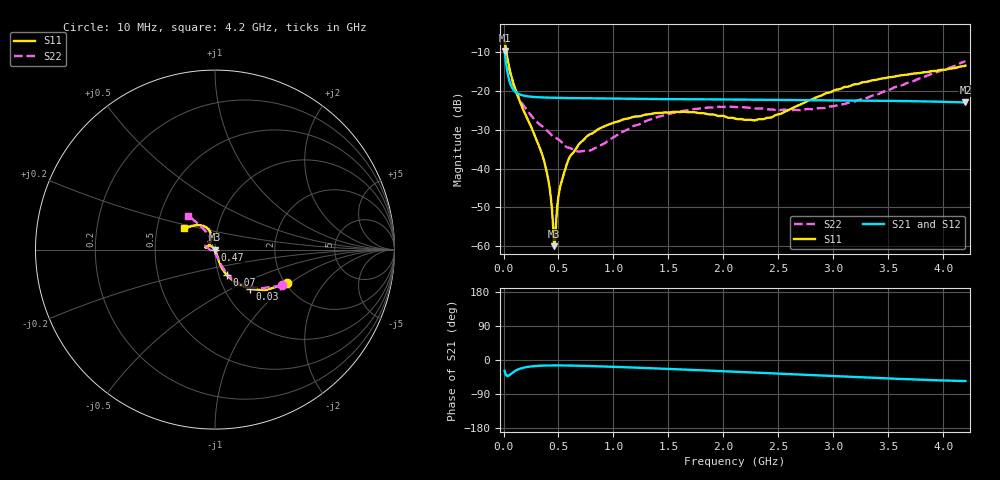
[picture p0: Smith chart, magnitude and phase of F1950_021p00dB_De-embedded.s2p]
! Integrated Device Technology
! Corporate Headquarters
! 6024 Silver Creek Valley Road
! San Jose, CA 95138  USA
! Phone:  1-408-284-8200
! Toll Free:  1-800-223-1366
! Webpage:  http://www.idt.com/
! Timing and RF Division
! 515 Groton Road, Suite 102
! Westford, MA 01886-6024
! Device:  F1950
! Description: 7-bit 0.25 dB Digital Step Attenuator
! Frequency:  150.0 -  4000.00 MHz
! Package:  4x4 mm Thin QFN Plastic Package: 24 pin
! Ports:  2 RF, 12 DC
!  Pin  1  = D0
!  Pin  2  = VDD
!  Pin  3  = Vmode
!  Pin  4  = GND
!  Pin  5  = RF1  =  Port 1
!  Pin  6  = GND
!  Pin  7  = GND
!  Pin  8  = GND
!  Pin  9  = GND
!  Pin 10  = GND
!  Pin 11  = GND
!  Pin 12  = GND
!  Pin 13  = GND
!  Pin 14  = RF2  =  Port 2
!  Pin 15  = GND
!  Pin 16  = LE
!  Pin 17  = CLK
!  Pin 18  = DATE
!  Pin 19  = D6
!  Pin 20  = D5
!  Pin 21  = D4
!  Pin 22  = D3
!  Pin 23  = D2
!  Pin 24  = D1
! State:  84
! Atten State:  21.00 dB
! Voltage:  +5.00 Volts
! Current:  Not Measured mA
! Data:  The device was measured on a the F195X evaluation board which has
!  individual transmission lines to the RF pins.  Data was collected
!  using a calibrated network analyzer.  The evaluation board was
!  de-embedded using a TRL calibration technique.
!  The reference plane is the edge of the package pin.
! Misc:  Board 2019
!  Action Tracker AT0250
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# GHz S dB R 50
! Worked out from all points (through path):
!   420 points, 10 MHz to 4.2 GHz, reference 50 ohm
!   highest |S21| = -9.63 dB at 10 MHz (marker M1); lowest = -23.0 dB at 4.2 GHz (marker M2)
!   group delay of S21, straight-line fit = 28.2 ps
!   lowest |S11| = -60.0 dB at 460 MHz (marker M3), VSWR 1.00, Z = 49.9 - j0.0787 ohm
!   |S11| at or under -10 dB: 26.17 MHz to end of sweep
!   |S22| runs from -35.6 to -7.5 dB; largest |S21 - S12| = 0.00013
!   S11 on the Smith chart (normalised r, x): 10 MHz: 2.05, -0.96; 30 MHz: 1.31, -0.63; 70 MHz: 1.09, -0.32; 470 MHz: 1.00, +0.00; 4.2 GHz: 0.69, +0.17
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0.01  -7.02 -24.9  -9.63 -28.4  -9.63 -28.4  -7.46 -28.1
0.03  -10.68 -48.4  -14.22 -41.8  -14.22 -41.8  -11.36 -49.2
0.07  -16.11 -64.9  -18.76 -36.1  -18.76 -36.1  -16.48 -63.5
0.16  -23.54 -71.3  -21.04 -22.1  -21.05 -22.1  -22.87 -70.7
0.36  -37.21 -66.5  -21.70 -14.8  -21.70 -14.8  -29.32 -77.6
0.41  -43.35 -70.8  -21.75 -14.4  -21.75 -14.4  -30.63 -78.7
0.45  -54.36 -90.9  -21.78 -14.3  -21.78 -14.3  -31.67 -83.3
0.46  -59.99 -128.1  -21.79 -14.3  -21.79 -14.3  -31.89 -84.8
0.47  -58.43 165.6  -21.80 -14.3  -21.80 -14.3  -32.05 -86.2
0.48  -52.92 145.1  -21.80 -14.3  -21.80 -14.3  -32.21 -87.3
0.51  -45.41 136.2  -21.82 -14.3  -21.82 -14.3  -32.74 -89.5
0.56  -40.31 133.0  -21.84 -14.5  -21.84 -14.5  -34.20 -95.5
0.61  -36.67 134.8  -21.86 -14.7  -21.86 -14.7  -34.77 -105.9
0.71  -33.10 136.8  -21.90 -15.3  -21.90 -15.3  -35.55 -125.6
0.99  -28.32 146.9  -21.99 -17.9  -21.99 -17.9  -32.14 -173.4
1.41  -25.71 163.0  -22.10 -22.5  -22.10 -22.5  -26.66 164.1
1.73  -25.49 168.4  -22.16 -26.2  -22.16 -26.2  -24.69 155.4
2.11  -27.16 157.9  -22.24 -31.1  -22.24 -31.1  -24.19 145.7
2.43  -26.87 125.9  -22.31 -35.0  -22.30 -35.0  -24.76 135.4
2.81  -22.13 105.0  -22.38 -40.0  -22.37 -40.0  -24.72 120.1
3.51  -16.49 117.2  -22.57 -48.8  -22.57 -48.8  -19.76 115.8
4.2  -13.52 145.7  -22.99 -55.5  -22.99 -55.6  -12.37 128.1
